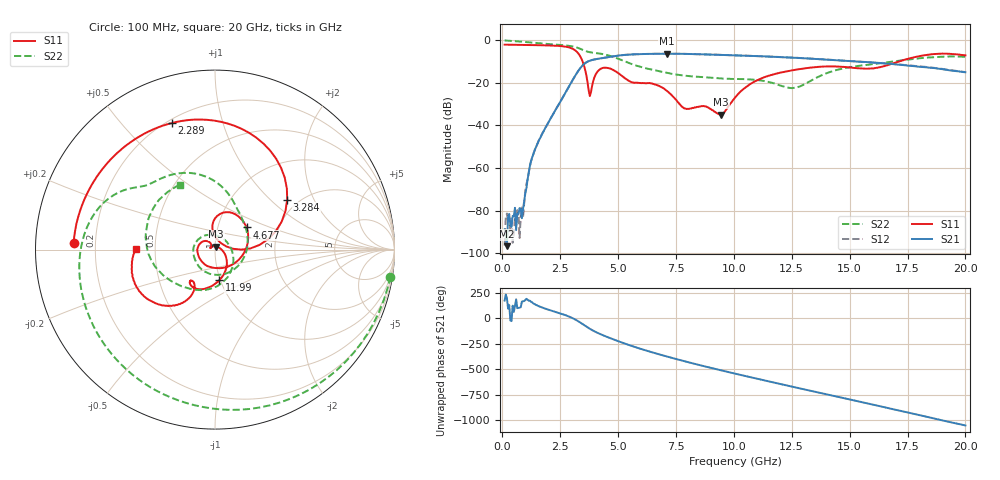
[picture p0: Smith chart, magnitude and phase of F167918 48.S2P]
!  2-Port S-parameters saved by WinCal
! VAR MeasName=S-Parameters (CALIBRATED_DATA) read from VNA (N5242A)
! VAR MeasDate=2016-11-22 10:27:07
! VAR NAME=F167918 48
! VAR FILENAME=F167918 48.S2P
! VAR DATE=2016-11-22 10:27:07
! VAR PHYS_PORTS=1,2
# Hz S DB R 50
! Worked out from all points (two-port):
!   401 points, 100 MHz to 20 GHz, reference 50 ohm
!   highest |S21| = -6.32 dB at 7.115 GHz (marker M1); lowest = -96.7 dB at 199.5 MHz (marker M2)
!   |S21| within 3 dB of the highest: 3.866 GHz to 14.31 GHz (10.44 GHz wide, 115 % of centre)
!   lowest |S11| = -34.9 dB at 9.453 GHz (marker M3), VSWR 1.04, Z = 50.6 + j1.71 ohm
!   |S11| at or under -10 dB: 3.469 GHz to 17.13 GHz (13.66 GHz wide, 133 % of centre)
!   |S22| runs from -22.5 to -0.1 dB; largest |S21 - S12| = 0.006
!   S11 on the Smith chart (normalised r, x): 100 MHz: 0.12, +0.02; 2.289 GHz: 0.22, +0.69; 3.284 GHz: 1.75, +1.28; 4.677 GHz: 1.37, +0.36; 11.99 GHz: 0.99, -0.35; 20 GHz: 0.39, +0.00
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1e8  -2.06 177.3  -88.80 174.5  -96.37 99.0  -0.10 -8.8
1.995e8  -2.07 174.6  -96.67 -161.7  -81.34 129.4  -0.16 -17.0
8.4625e8  -2.17 157.3  -83.56 164.1  -78.53 144.9  -0.68 -67.1
1.34375e9  -2.26 143.1  -53.35 145.6  -53.35 145.9  -1.21 -100.4
2.289e9  -2.56 109.0  -32.88 64.5  -32.89 63.9  -2.02 -153.1
3.284e9  -6.22 34.6  -14.33 -29.0  -14.35 -29.0  -3.65 154.2
3.43325e9  -9.03 16.8  -12.22 -50.9  -12.22 -50.8  -4.32 147.2
3.7815e9  -26.22 49.0  -9.59 -102.5  -9.56 -102.6  -5.62 136.8
4.1795e9  -13.97 82.0  -8.64 -149.2  -8.62 -149.4  -6.20 123.4
4.677e9  -13.35 35.1  -7.72 164.1  -7.72 164.0  -7.40 101.6
5.62225e9  -19.79 -90.1  -6.63 86.7  -6.61 86.6  -11.33 65.3
6.7665e9  -21.40 150.4  -6.34 7.6  -6.36 7.4  -14.52 14.3
7.11475e9  -23.84 132.9  -6.32 -14.5  -6.34 -14.6  -15.32 -7.9
8.259e9  -31.80 162.0  -6.48 -83.5  -6.50 -83.4  -17.02 -87.2
9.453e9  -34.88 69.7  -6.85 -149.8  -6.87 -149.8  -17.95 -142.9
1.005e10  -26.93 -10.9  -7.06 178.1  -7.08 178.2  -18.21 -161.4
1.199025e10  -15.24 -81.8  -7.93 77.3  -7.87 77.3  -21.22 107.3
1.338325e10  -12.79 -106.7  -8.68 6.0  -8.62 6.0  -18.67 -28.3
1.507475e10  -12.85 -128.0  -9.82 -78.6  -9.79 -78.9  -12.55 -107.0
1.67165e10  -11.44 -117.1  -11.02 -162.4  -11.01 -162.4  -10.21 -148.0
1.835825e10  -6.85 -140.3  -12.76 113.4  -12.58 113.0  -8.11 169.8
2e10  -7.09 179.5  -15.02 29.9  -14.96 29.1  -7.76 118.3
